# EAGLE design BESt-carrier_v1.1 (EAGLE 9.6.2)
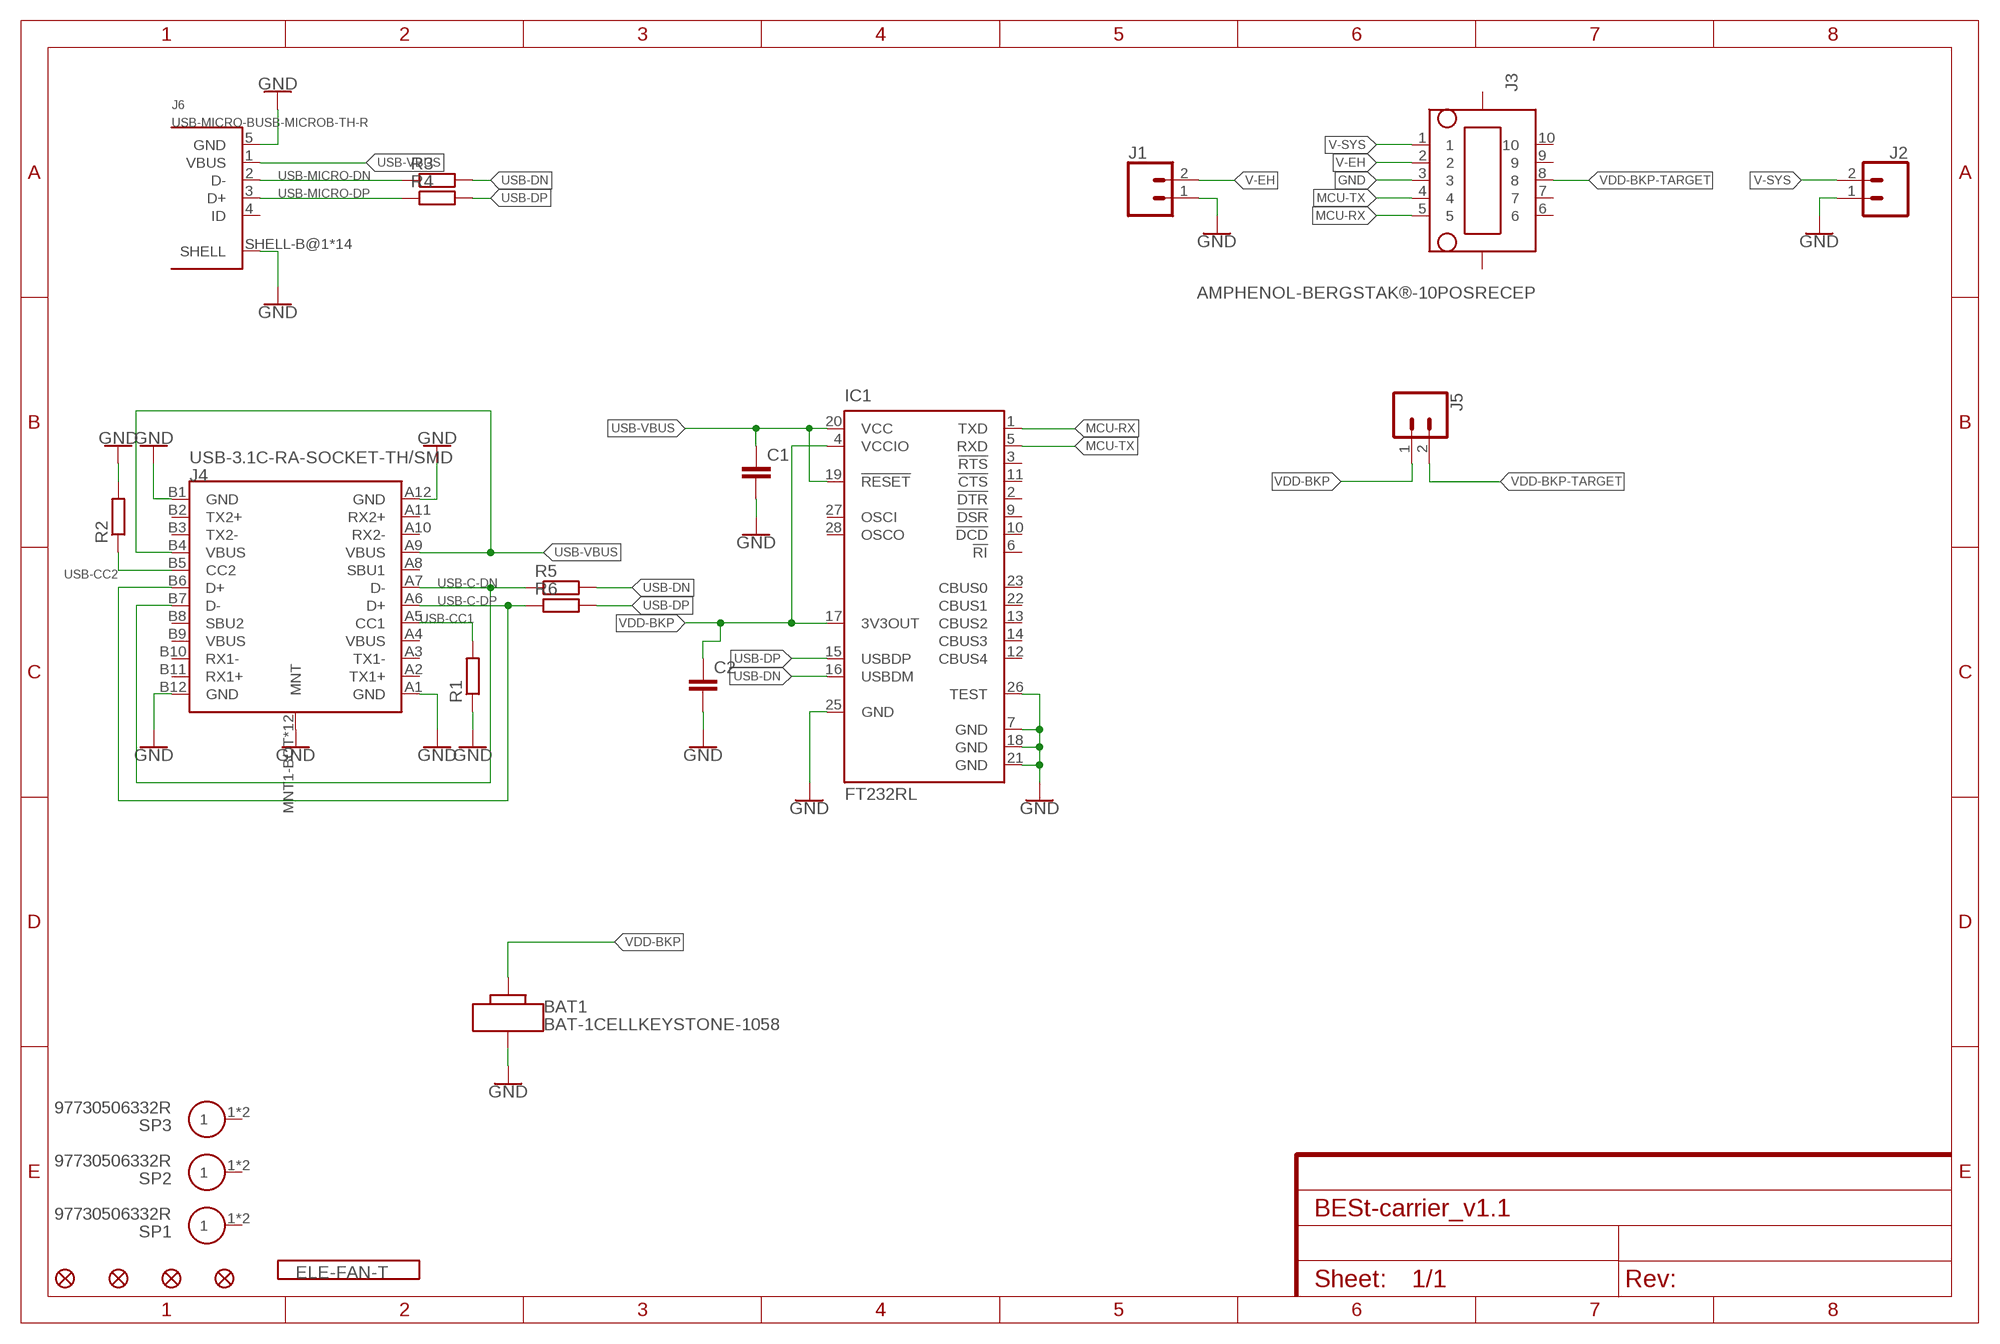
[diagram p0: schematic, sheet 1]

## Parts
BAT1  BAT-1CELLKEYSTONE-1058  [KEYSTONE-1058]
C1  C-EUC0603  [C0603]
C2  C-EUC0603  [C0603]
FD1  FIDUCIAL1X2  [FIDUCIAL-1X2]
FD2  FIDUCIAL1X2  [FIDUCIAL-1X2]
FD3  FIDUCIAL1X2  [FIDUCIAL-1X2]
FD4  FIDUCIAL1X2  [FIDUCIAL-1X2]
IC1  FT232RL  [SSOP28]
J1  CONN_025MM  [SCREWTERMINAL-5MM-2]
J2  CONN_025MM  [SCREWTERMINAL-5MM-2]
J3  AMPHENOL-BERGSTAK®-10POSRECEP  [10132798-10POS-RECEP]
J4  USB-3.1C-RA-SOCKET-TH/SMD  [GCT-USB4065-30-A]
J5  CONN_02  [1X02]
J6  USB-MICRO-BUSB-MICROB-TH-R  [AMPHENOL-10118194]
LOGO1  ELE-FAN-T  [ELE-FAN-T]
R1  R-EU_R0603  [R0603]
R2  R-EU_R0603  [R0603]
R3  R-EU_R0402  [R0402]
R4  R-EU_R0402  [R0402]
R5  R-EU_R0402  [R0402]
R6  R-EU_R0402  [R0402]
SP1  97730506332R  [M1.6]
SP2  97730506332R  [M1.6]
SP3  97730506332R  [M1.6]

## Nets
GND: BAT1.N C1.2 C2.2 IC1.7(GND) IC1.18(GND) IC1.21(GND) IC1.25(GND) IC1.26(TEST) J1.1 J2.1 J3.3 J4.A1(GND) J4.A12(GND) J4.B1(GND) J4.B12(GND) J4.MNT1-BOT(MNT) J4.MNT1-TH(MNT) J4.MNT1-TOP(MNT) J4.MNT2-BOT(MNT) J4.MNT2-TH(MNT) J4.MNT2-TOP(MNT) J4.MNT3-BOT(MNT) J4.MNT3-TH(MNT) J4.MNT3-TOP(MNT) J4.MNT4-BOT(MNT) J4.MNT4-TH(MNT) J4.MNT4-TOP(MNT) J6.5(GND) J6.SHELL-B@1(SHELL) J6.SHELL-B@2(SHELL) J6.SHELL@1-B(SHELL) J6.SHELL@1-T(SHELL) J6.SHELL@1-TH(SHELL) J6.SHELL@2-B(SHELL) J6.SHELL@2-T(SHELL) J6.SHELL@2-TH(SHELL) J6.SHELL@3-B(SHELL) J6.SHELL@3-T(SHELL) J6.SHELL@3-TH(SHELL) J6.SHELL@4-B(SHELL) J6.SHELL@4-T(SHELL) J6.SHELL@4-TH(SHELL) R1.1 R2.2
MCU-RX: IC1.1(TXD) J3.5
MCU-TX: IC1.5(RXD) J3.4
USB-C-DN: J4.A7(D-) J4.B7(D-) R5.1
USB-C-DP: J4.A6(D+) J4.B6(D+) R6.1
USB-CC1: J4.A5(CC1) R1.2
USB-CC2: J4.B5(CC2) R2.1
USB-DN: IC1.16(USBDM) R3.2 R5.2
USB-DP: IC1.15(USBDP) R4.2 R6.2
USB-MICRO-DN: J6.2(D-) R3.1
USB-MICRO-DP: J6.3(D+) R4.1
USB-VBUS: C1.1 IC1.19(!RESET) IC1.20(VCC) J4.A9(VBUS) J4.B4(VBUS) J6.1(VBUS)
V-EH: J1.2 J3.2
V-SYS: J2.2 J3.1
VDD-BKP: BAT1.P C2.1 IC1.4(VCCIO) IC1.17(3V3OUT) J5.1
VDD-BKP-TARGET: J3.8 J5.2
Unconnected: IC1.2(!DTR) IC1.3(!RTS) IC1.6(!RI) IC1.9(!DSR) IC1.10(!DCD) IC1.11(!CTS) IC1.12(CBUS4) IC1.13(CBUS2) IC1.14(CBUS3) IC1.22(CBUS1) IC1.23(CBUS0) IC1.27(OSCI) IC1.28(OSCO) J3.6 J3.7 J3.9 J3.10 J3.MNT1 J3.MNT2 J4.A2(TX1+) J4.A3(TX1-) J4.A4(VBUS) J4.A8(SBU1) J4.A10(RX2-) J4.A11(RX2+) J4.B2(TX2+) J4.B3(TX2-) J4.B8(SBU2) J4.B9(VBUS) J4.B10(RX1-) J4.B11(RX1+) J6.4(ID) SP1.1 SP1.1T SP2.1 SP2.1T SP3.1 SP3.1T

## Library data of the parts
BAT1 = Fan_Battery_Holder:BAT-1CELL
C1 C2 = rcl:C-EU: CAPACITOR, European symbol; SPICEPREFIX: C
FD1-FD4 = SparkFun-Aesthetics:FIDUCIAL: Fiducial Alignment Points
IC1 = ftdichip:FT232R: Source: http://www.ftdichip.com/Documents/DataSheets/DS_FT232R_v104.pdf; MPN: FT232RL; OC_FARNELL: 1146032; OC_NEWARK: 91K9918
J1 J2 = SparkFun-Connectors:CONN_02: Multi connection point. Often used as Generic Header-pin footprint for 0.1 inch spaced/style header connections; SF_SKU: PRT-08432
J3 = Fan_B2B_connector:AMPHENOL-BERGSTAK®-10POS: Amphenol’s BergStak® 0.5mm is a comprehensive and versatile board-to-board solution designed for reliable and high-density applications. The unique design of scoop-proof housing ensures terminals are not damaged during mating.
J4 = Fan_Connectors:USB-3.1
J5 = SparkFun-Connectors:CONN_02: Multi connection point. Often used as Generic Header-pin footprint for 0.1 inch spaced/style header connections
J6 = Fan_Connectors:USB-MICRO-B
LOGO1 = Fan_logo:ELE-FAN-T
R1-R6 = rcl:R-EU_: RESISTOR, European symbol; SPICEPREFIX: R
SP1-SP3 = Fan_Spacer:97730506332R: M1.6, Round Female, 5 mm, WA-SMSI Series

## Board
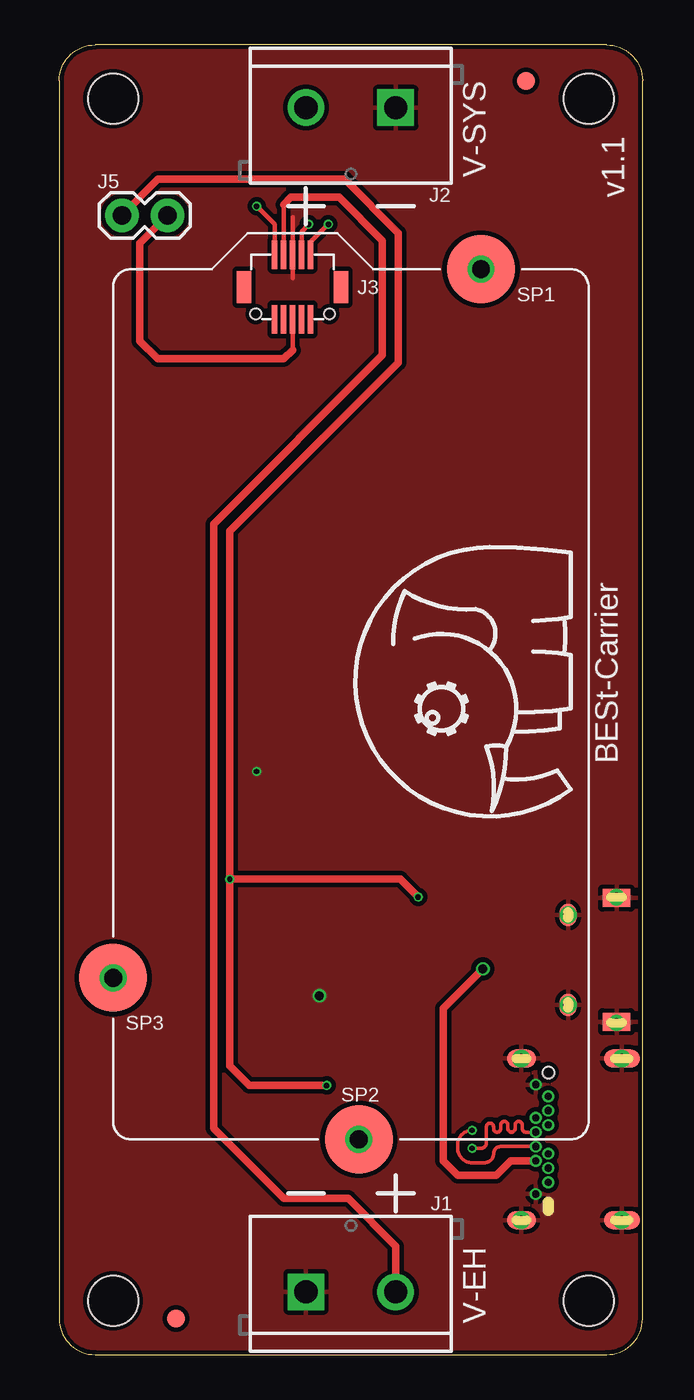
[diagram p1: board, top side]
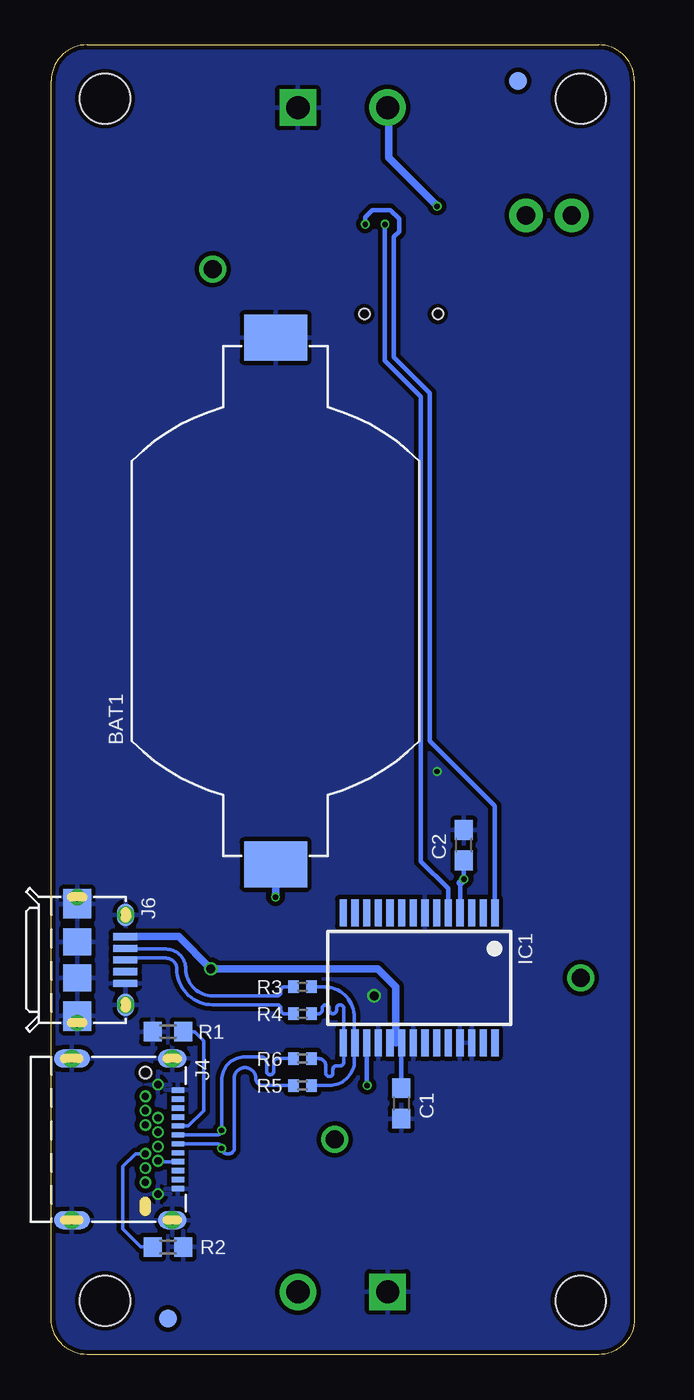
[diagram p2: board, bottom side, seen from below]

Size 32.5 x 73 mm. Coordinates in mm from the lower left corner, seen from the top.
Outline: 2,0 30.5,0 arc90 32.5,2 32.5,71 arc90 30.5,73 2,73 arc90 0,71 0,2 arc90 2,0
Copper layers (1*16): Top 0.035mm / dielectric 1.5mm / Bottom 0.035mm
Design rules "SparkFun *": minimum track width 0.2mm, minimum drill 0.3mm, track to track 6mil, track to pad 6mil, pad to pad 0.15mm, via to via 6mil, smd to smd 0mil, copper to edge 6mil, drill to drill 6mil, minimum pad ring 0.125mm, minimum via ring 0.1mm, stop-mask expansion 4mil, vias tented up to drill 25mil, thermal gap 10mil
Holes 2.8 mm at 3,3 29.5,3 29.5,70 3,70

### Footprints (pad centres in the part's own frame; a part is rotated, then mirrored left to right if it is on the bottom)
KEYSTONE-1058 = smd 2.54 x 3.51: N 14.68,0; P -14.68,0
C0603 = smd 1.1 x 1: 1 -0.85,0; 2 0.85,0
FIDUCIAL-1X2 = smd 1 x 1: 1 0,0
SSOP28 = smd 0.4 x 1.5: 1 -4.225,-3.625; 2 -3.575,-3.625; 3 -2.925,-3.625; 4 -2.275,-3.625; 5 -1.625,-3.625; 6 -0.975,-3.625; 7 -0.325,-3.625; 8 0.325,-3.625; 9 0.975,-3.625; 10 1.625,-3.625; 11 2.275,-3.625; 12 2.925,-3.625; 13 3.575,-3.625; 14 4.225,-3.625; 15 4.225,3.625; 16 3.575,3.625; 17 2.925,3.625; 18 2.275,3.625; 19 1.625,3.625; 20 0.975,3.625; 21 0.325,3.625; 22 -0.325,3.625; 23 -0.975,3.625; 24 -1.625,3.625; 25 -2.275,3.625; 26 -2.925,3.625; 27 -3.575,3.625; 28 -4.225,3.625
SCREWTERMINAL-5MM-2 = drill 1.3 pad 2.032 square: 1 0,0 | drill 1.3 pad 2.032: 2 5,0
10132798-10POS-RECEP = smd 0.3 x 1.6: 1 -1,1.8; 2 -0.5,1.8; 3 0,1.8; 4 0.5,1.8; 5 1,1.8; 6 1,-1.8; 7 0.5,-1.8; 8 0,-1.8; 9 -0.5,-1.8; 10 -1,-1.8 | smd 0.8 x 1.8: MNT1 -2.7,0; MNT2 2.7,0 | hole 0.6: -2.05,-1.5; 2.05,-1.5
GCT-USB4065-30-A = smd 0.3 x 0.7: A1 -2.75,7.06; A2 -2.25,7.06; A3 -1.75,7.06; A4 -1.25,7.06; A5 -0.75,7.06; A6 -0.25,7.06; A7 0.25,7.06; A8 0.75,7.06; A9 1.25,7.06; A10 1.75,7.06; A11 2.25,7.06; A12 2.75,7.06 | drill 0.4 pad 0.65: B1 3.05,5.95; B2 2.4,5.25; B3 1.6,5.25; B4 1.2,5.95; B5 0.8,5.25; B6 0.4,5.95; B7 -0.4,5.95; B8 -0.8,5.25; B9 -1.2,5.95; B10 -1.6,5.25; B11 -2.4,5.25; B12 -3.05,5.95 | smd 1 x 2 bottom: MNT1-BOT -4.5,1.15; MNT2-BOT 4.5,1.15 | drill 0.5 pad 1: MNT1-TH -4.5,1.15; MNT2-TH 4.5,1.15; MNT3-TH -4.5,6.75; MNT4-TH 4.5,6.75 | smd 1 x 2: MNT1-TOP -4.5,1.15; MNT2-TOP 4.5,1.15 | smd 1 x 1.6 bottom: MNT3-BOT -4.5,6.75; MNT4-BOT 4.5,6.75 | smd 1 x 1.6: MNT3-TOP -4.5,6.75; MNT4-TOP 4.5,6.75 | hole 0.65: -3.725,5.25
1X02 = drill 1.016 pad 1.88: 1 0,0; 2 2.54,0
AMPHENOL-10118194 = smd 0.4 x 1.35: 1 -1.3,4.125; 2 -0.65,4.125; 3 0,4.125; 4 0.65,4.125; 5 1.3,4.125 | smd 1.5 x 1.55: SHELL-B@1 -1,1.45; SHELL-B@2 1,1.45 | smd 1.25 x 0.95 bottom: SHELL@1-B -2.5,4.15; SHELL@2-B 2.5,4.15 | smd 1.25 x 0.95: SHELL@1-T -2.5,4.15; SHELL@2-T 2.5,4.15 | drill 0.55 pad 0.95: SHELL@1-TH -2.5,4.15; SHELL@2-TH 2.5,4.15 | smd 1 x 1.55 bottom: SHELL@3-B -3.45,1.45; SHELL@4-B 3.45,1.45 | smd 1.65 x 1.55: SHELL@3-T -3.125,1.45; SHELL@4-T 3.125,1.45 | drill 0.5 pad 0.9: SHELL@3-TH -3.5,1.45; SHELL@4-TH 3.5,1.45
R0603 = smd 1 x 1.1: 1 -0.85,0; 2 0.85,0
R0402 = smd 0.6 x 0.7: 1 -0.5,0; 2 0.5,0
M1.6 = drill 1: 1 0,0 | smd 3.8 x 3.8: 1T 0,0

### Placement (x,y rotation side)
BAT1  20,42 90 bottom
C1  13,14 270 bottom
C2  9.5,28.4 90 bottom
FD1  6.5,2 0 top
FD2  26,71 0 top
FD3  26,2 0 bottom
FD4  6.5,71 0 bottom
IC1  12,21 180 bottom
J1  13.75,3.5 0 top
J2  18.75,69.5 180 top
J3  13,59.5 0 top
J4  32.5,12 270 bottom
J5  3.5,63.5 0 top
J6  32.5,22 270 bottom
LOGO1  28.5,30 90 top
R1  26,18 0 bottom
R2  26,6 0 bottom
R3  18.5,20.5 0 bottom
R4  18.5,19 0 bottom
R5  18.5,15 0 bottom
R6  18.5,16.5 0 bottom
SP1  23.5,60.5 0 top
SP2  16.7,12 0 top
SP3  3,21 0 top

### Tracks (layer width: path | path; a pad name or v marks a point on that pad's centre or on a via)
GND  (via drill 0.3, 0.5)
  Top 0.254: 13,60 J3.3 13,63.4
  other vias: 11,32.5 14.5,20
  pour Top (isolate 0.254, rank 6): 0,0 0,73 32.5,73 32.5,0
  pour Bottom (isolate 0.254, rank 6): 0,0 0,73 32.5,73 32.5,0
MCU-RX  (via drill 0.3)
  Top 0.254: J3.5 14,62 v15,63
  Bottom 0.254: v15,63 15,63.4 14.6,63.8 13.6,63.8 13.1,63.3 13.1,62.6 13.4,62.3 13.4,55.6 11.4,53.6 11.4,34.2 7.78,30.57 IC1.1
MCU-TX  (via drill 0.3)
  Top 0.254: v13.9,63 13.5,62.6 J3.4
  Bottom 0.254: v13.9,63 13.9,55.4 11.9,53.4 11.9,27.5 10.38,25.98 IC1.5
USB-C-DN  (via drill 0.3)
  Top 0.2: J4.B7 26,12.4 arc-90 25.8,12.6 25.8,12.8 arc90 25.6,13 arc90 25.4,12.8 25.4,12.6 arc-90 25.2,12.4 arc-90 25,12.6 25,12.8 arc90 24.8,13 arc90 24.6,12.8 24.6,12.6 arc-90 24.4,12.4 arc-90 24.2,12.6 24.2,12.7 arc90 24,12.9 arc90 23.8,12.7 23.8,11.8 arc-90 23.5,11.5 v23,11.5
  Bottom 0.2: J4.A7 23.25,11.75 arc90 v23,11.5 arc-90 22.7,11.2 22.6,11.2 arc-90 22.3,11.5 22.3,15.4 arc90 21.7,16 arc90 21.1,15.4 arc-90 20.7,15 R5.1
USB-C-DP  (via drill 0.3)
  Top 0.2: v23,12.5 arc90 22.2,11.7 22.2,11.5 arc90 23,10.7 23.7,10.7 arc90 24.2,11.2 arc-90 24.6,11.6 J4.B6
  Bottom 0.2: J4.A6 23.25,12.25 arc-90 v23,12.5 23,15.3 arc90 21.7,16.6 20.8,16.6 arc90 20.5,16.3 20.5,15.8 arc-90 20.3,15.6 arc-90 20.1,15.8 20.1,16.3 arc90 19.9,16.5 R6.1
USB-CC1
  Bottom 0.2: J4.A5 24.85,12.75 24,13.6 24,17.5 24.5,18 R1.2
USB-CC2
  Bottom 0.2: J4.B5 27.8,11.2 28.5,10.5 28.5,7 27.5,6 R2.1
USB-DN
  Bottom 0.2: R3.2 17.3,20.5 arc90 15.6,18.8 15.6,17.4 arc-90 IC1.16 arc-90 15.6,17.35 15.6,16.4 arc90 17,15 R5.2
  Bottom 0.254: IC1.16 15.6,17.35
USB-DP
  Bottom 0.2: R4.2 17.6,19 arc-90 17.4,19.2 17.4,19.3 arc90 17.2,19.5 arc90 17,19.3 17,19.2 arc-90 16.8,19 arc-90 16.6,19.2 16.6,19.3 arc90 16.4,19.5 arc90 16.2,19.3 16.2,17.4 | 16.2,17.4 arc90 IC1.15 | R6.2 17.6,16.5 arc90 17.2,16.1 17.2,15.7 arc-90 17,15.5 arc-90 16.8,15.7 16.8,15.9 arc90 16.6,16.1 16.4,16.1 arc-90 16.2,16.3 16.2,17.4
USB-MICRO-DN
  Bottom 0.2: R3.1 19.5,20.5 arc-90 19.7,20.3 19.7,20.2 arc90 19.9,20 23.5,20 arc90 25,21.5 arc-90 26.1,22.6 28.32,22.6 J6.2
USB-MICRO-DP
  Bottom 0.2: R4.1 19.5,19 arc90 19.7,19.2 19.7,19.3 arc-90 19.9,19.5 23.5,19.5 arc90 25.5,21.5 arc-90 26.1,22.1 28.27,22.1 J6.3
USB-VBUS  (via drill 0.5)
  Top 0.406: v23.6,21.5 21.4,19.3 21.4,10.8 22.2,10 24.35,10 25.15,10.8 J4.B4
  Bottom 0.2: J4.A9 26.5,10.75 J4.B4
  Bottom 0.254: IC1.19 13.3,17.38 IC1.20 13,17.35 C1.1
  Bottom 0.406: 13.3,17.38 13.3,20.5 14.3,21.5 v23.6,21.5 25.4,23.3 J6.1
V-EH
  Top 0.254: 12.5,64.1 J3.2
  Top 0.406: J1.2 18.75,6.05 16.1,8.7 12.5,8.7 8.6,12.6 8.6,46.3 18,55.7 18,62.1 15.6,64.5 12.9,64.5 12.5,64.1
V-SYS  (via drill 0.3)
  Top 0.254: J3.1 12,63 v11,64
  Bottom 0.406: v11,64 13.7,66.7 13.7,69.45 J2.2
VDD-BKP  (via drill 0.3)
  Top 0.406: v14.9,15 10.6,15 9.5,16.1 v9.5,26.5 | v20,25.5 19,26.5 v9.5,26.5 | v9.5,26.5 9.5,45.9 18.9,55.3 18.9,62.5 15.9,65.5 5.5,65.5 J5.1
  Bottom 0.254: IC1.17 14.93,15.03 v14.9,15 | IC1.4 9.7,24.65 9.7,26.3 | C2.1 v9.5,26.5
  Bottom 0.406: v9.5,26.5 9.7,26.3 | BAT1.P v20,25.5
VDD-BKP-TARGET
  Top 0.254: J3.8 13,56
  Top 0.406: 13,56 12.5,55.5 5.5,55.5 4.5,56.5 4.5,61.96 J5.2

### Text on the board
tNames: V-SYS | v1.1 | BESt-Carrier | V-EH

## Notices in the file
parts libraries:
SparkFun-Connectors: Licensing: Creative Commons ShareAlike 4.0 International - https://creativecommons.org/licenses/by-sa/4.0
